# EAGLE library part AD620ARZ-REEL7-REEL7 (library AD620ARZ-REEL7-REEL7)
Check availability
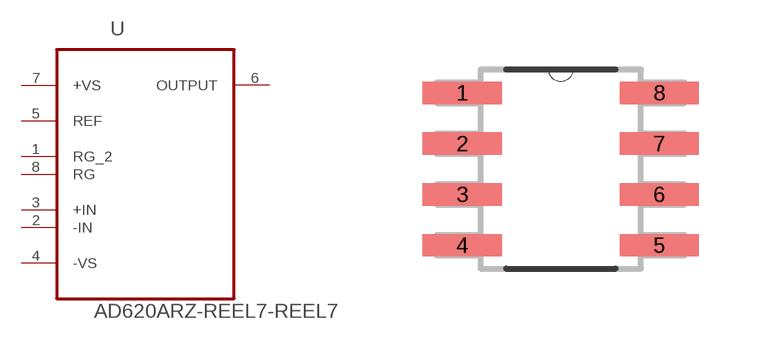
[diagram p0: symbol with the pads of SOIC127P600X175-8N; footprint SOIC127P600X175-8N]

Designator prefix U

## AD620ARZ-REEL7-REEL7 (Availability: In Stock; Check_prices: https://www.snapeda.com/parts/AD620ARZ-REEL7/Analog+Devices/view-part/?ref=eda; Description: Low Drift, Low Power Instrumentation Amp with Set Gains of 1 to 10000; MF: Analog Devices; MP: AD620ARZ-REEL7; Package: SOIC-8 Analog Devices; Price: None; Purchase-URL: https://www.snapeda.com/api/url_track_click_mouser/?unipart_id=48261&manufacturer=Analog Devices&part_name=AD620ARZ-REEL7&search_term=ad620; SnapEDA_Link: https://www.snapeda.com/parts/AD620ARZ-REEL7/Analog+Devices/view-part/?ref=snap)  [SOIC127P600X175-8N]
1  RG_2  pas
2  -IN  in
3  +IN  in
4  -VS  pwr
5  REF  pas
6  OUTPUT  out
7  +VS  pwr
8  RG  pas

## Footprint SOIC127P600X175-8N (pad centres in mm)
smd 1.981 x 0.559: 1 -2.464,1.905; 2 -2.464,0.635; 3 -2.464,-0.635; 4 -2.464,-1.905; 5 2.464,-1.905; 6 2.464,-0.635; 7 2.464,0.635; 8 2.464,1.905

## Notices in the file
This work is licensed under a Creative Commons Attribution-ShareAlike 4.0 International License (CC BY-SA) with Design Exception 1.0
